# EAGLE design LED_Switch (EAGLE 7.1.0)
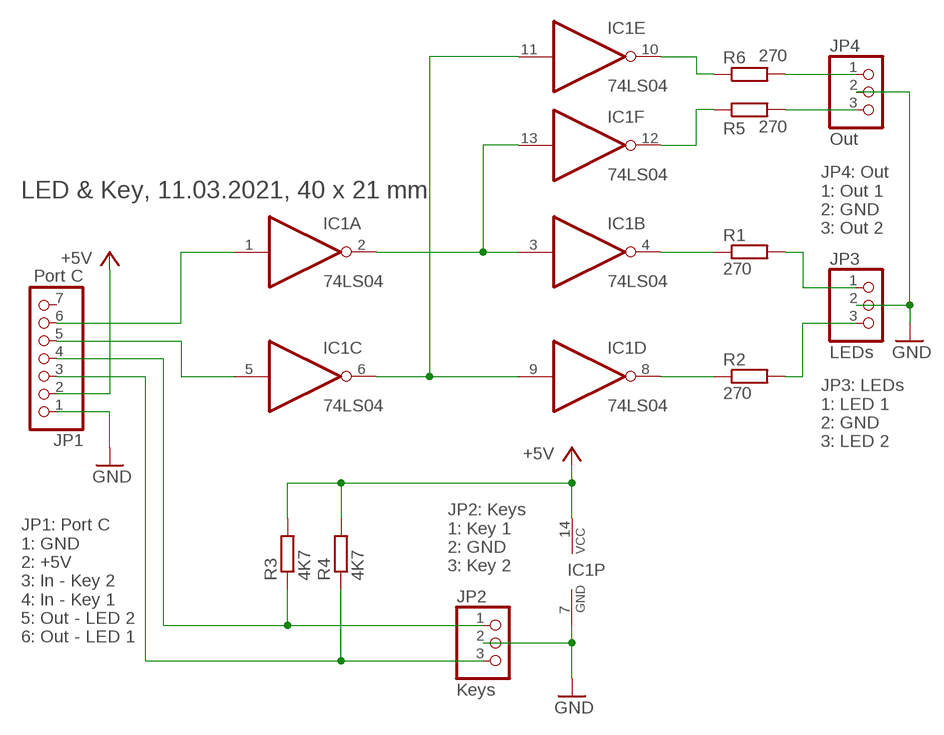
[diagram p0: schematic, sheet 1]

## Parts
IC1  74LS04  74ACT04D  [SO14]
JP1  Port C  PINHD-1X7  [1X07]
JP2  Keys  PINHD-1X3  [1X03]
JP3  LEDs  PINHD-1X3  [1X03]
JP4  Out  PINHD-1X3  [1X03]
R1  270  R-EU_R1206  [R1206]
R2  270  R-EU_R1206  [R1206]
R3  4K7  R-EU_R1206  [R1206]
R4  4K7  R-EU_R1206  [R1206]
R5  270  R-EU_R1206  [R1206]
R6  270  R-EU_R1206  [R1206]

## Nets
+5V: IC1.14(P:VCC) JP1.2 R3.2 R4.2
GND: IC1.7(P:GND) JP1.1 JP2.2 JP3.2 JP4.2
N$1: IC1.2(A:O) IC1.3(B:I) IC1.13(F:I)
N$2: IC1.6(C:O) IC1.9(D:I) IC1.11(E:I)
N$3: IC1.1(A:I) JP1.6
N$4: IC1.5(C:I) JP1.5
N$5: IC1.4(B:O) R1.1
N$6: IC1.8(D:O) R2.1
N$7: IC1.10(E:O) R6.1
N$8: JP3.1 R1.2
N$9: JP1.4 JP2.1 R3.1
N$10: JP1.3 JP2.3 R4.1
N$11: JP3.3 R2.2
N$12: IC1.12(F:O) R5.1
N$15: JP4.1 R6.2
N$16: JP4.3 R5.2
Unconnected: JP1.7

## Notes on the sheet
- LED & Key, 11.03.2021, 40 x 21 mm
- JP4: Out
  1: Out 1
  2: GND
  3: Out 2
- JP3: LEDs
  1: LED 1
  2: GND
  3: LED 2
- JP2: Keys
  1: Key 1
  2: GND
  3: Key 2
- JP1: Port C
  1: GND
  2: +5V
  3: In - Key 2
  4: In - Key 1
  5: Out - LED 2
  6: Out - LED 1

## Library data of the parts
IC1 = 74xx-eu:74*04: Hex INVERTER
JP1 = pinhead:PINHD-1X7: PIN HEADER
JP2-JP4 = pinhead:PINHD-1X3: PIN HEADER
R1-R6 = rcl:R-EU_: RESISTOR, European symbol

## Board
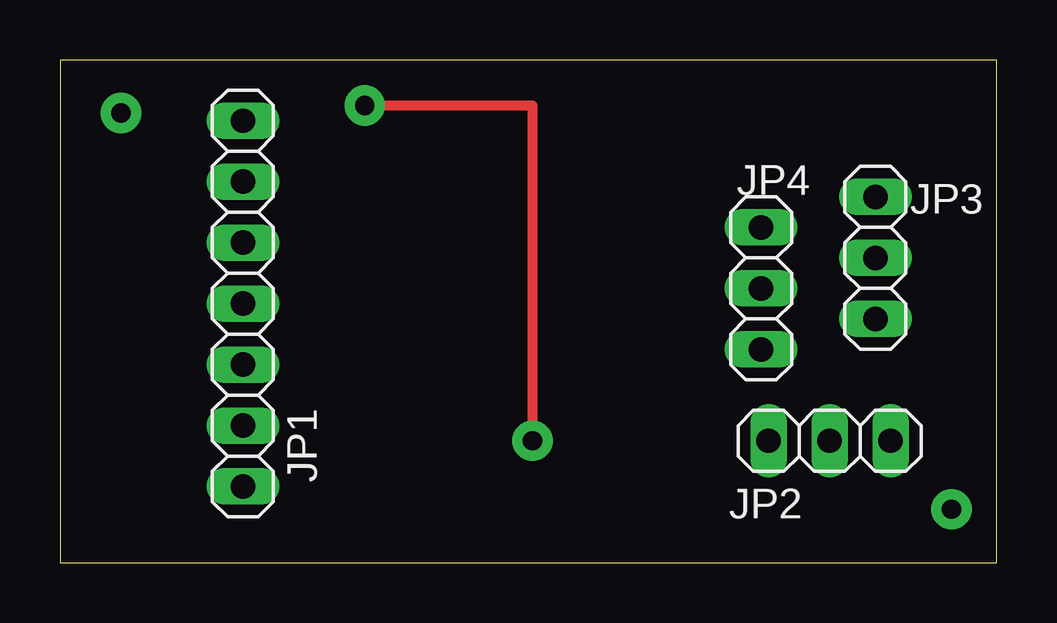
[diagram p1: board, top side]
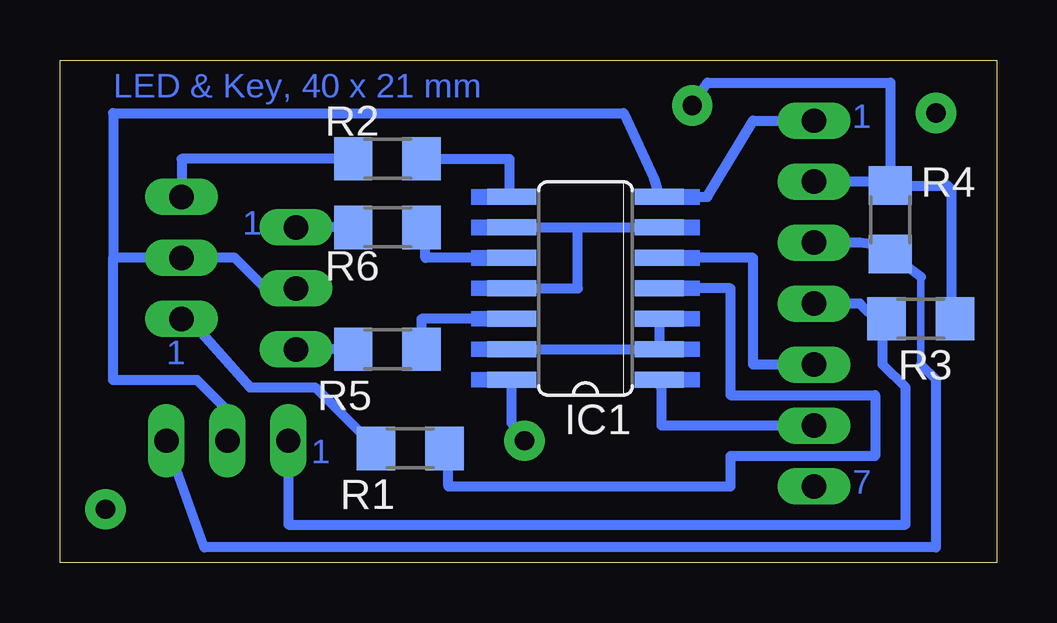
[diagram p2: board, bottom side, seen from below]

Size 39.04 x 20.95 mm. Coordinates in mm from the lower left corner, seen from the top.
Outline: 0,0 39.04,0 39.04,20.95 0,20.95 0,0
Copper layers (1*16): Top 0.035mm / dielectric 1.5mm / Bottom 0.035mm
Design rules "default": minimum track width 10mil, minimum drill 24mil, track to track 8mil, track to pad 8mil, pad to pad 8mil, via to via 8mil, smd to smd 8mil, copper to edge 40mil, drill to drill 8mil, minimum pad ring 10mil, minimum via ring 8mil, stop-mask expansion 4mil, vias tented up to drill 0mil, thermal gap 10mil

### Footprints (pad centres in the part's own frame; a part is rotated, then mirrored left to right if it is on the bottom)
SO14 = smd 0.66 x 2.032: 1 -3.81,-3.073; 2 -2.54,-3.073; 3 -1.27,-3.073; 4 0,-3.073; 5 1.27,-3.073; 6 2.54,-3.073; 7 3.81,-3.073; 8 3.81,3.073; 9 2.54,3.073; 10 1.27,3.073; 11 0,3.073; 12 -1.27,3.073; 13 -2.54,3.073; 14 -3.81,3.073
1X07 = drill 1.016 long: 1 -7.62,0; 2 -5.08,0; 3 -2.54,0; 4 0,0; 5 2.54,0; 6 5.08,0; 7 7.62,0
1X03 = drill 1.016 long: 1 -2.54,0; 2 0,0; 3 2.54,0
R1206 = smd 1.6 x 1.803: 1 -1.422,0; 2 1.422,0

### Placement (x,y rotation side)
IC1  17.14,11.43 90 bottom
JP1  7.62,10.79 270 top
JP2  32.07,5.08 0 top
JP3  33.97,12.7 90 top
JP4  29.21,11.43 270 top
R1  24.45,4.76 180 bottom
R2  25.4,16.83 180 bottom
R3  3.17,10.16 0 bottom
R4  4.45,14.29 90 bottom
R5  25.4,8.89 180 bottom
R6  25.4,13.97 180 bottom

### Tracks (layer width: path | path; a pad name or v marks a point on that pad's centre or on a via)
+5V  (via drill 0.8 pad 1.68)
  Top 0.406: v12.7,19.05 19.68,19.05 v19.68,5.08
  Bottom 0.406: R3.2 1.91,10.31 1.91,15.56 2.06,15.71 R4.2 4.45,15.88 | v19.68,5.08 20.22,5.82 IC1.14 | v12.7,19.05 12.06,20 4.45,20 4.45,15.88 | 4.45,15.88 JP1.2
GND
  Bottom 0.406: 36.83,12.7 JP3.2 31.75,12.7 30.48,11.43 JP4.2 | JP1.1 10.16,18.41 12.06,15.24 IC1.7 14.29,15.98 15.56,18.73 36.83,18.73 36.83,12.7 | 36.83,12.7 36.83,7.62 33.34,7.62 32.07,6.35 JP2.2
N$1
  Bottom 0.406: IC1.3 IC1.2 IC1.13
N$2
  Bottom 0.406: IC1.9 17.46,13.97 | 17.46,13.97 IC1.6 | IC1.11 17.46,11.43 17.46,13.97
N$3
  Bottom 0.406: 14.07,7.4 IC1.1 13.97,7.52 13.97,5.71 JP1.6
N$4
  Bottom 0.406: JP1.5 10.16,8.26 10.16,12.7 IC1.5
N$5
  Bottom 0.406: IC1.4 11.11,11.43 11.11,6.99 5.08,6.99 5.08,4.45 11.11,4.45 11.11,3.17 22.86,3.17 22.86,4.6 R1.1
N$6
  Bottom 0.406: IC1.8 20.32,15.24 20.32,16.83 R2.1
N$7
  Bottom 0.406: IC1.10 23.81,12.7 23.81,13.97 R6.1
N$8
  Bottom 0.406: JP3.1 33.66,10.16 31.11,7.3 28.41,7.3 R1.2
N$9
  Bottom 0.406: R3.1 4.45,10.16 | JP2.1 29.53,1.59 3.81,1.59 3.81,7.3 4.76,8.26 4.76,9.99 R3.1 | R3.1 4.92,9.99 5.71,10.79 JP1.4
N$10
  Bottom 0.305: 3.17,8.26 3.17,11.91
  Bottom 0.406: 3.17,8.26 2.54,7.62 2.54,0.64 33.02,0.64 JP2.3 | 3.17,11.91 R4.1 4.61,13.18 5.71,13.34 JP1.3
N$11
  Bottom 0.406: R2.2 33.97,16.83 JP3.3
N$12
  Bottom 0.406: IC1.12 23.98,10.16 R5.1
N$13  (via drill 0.8 pad 1.68)
  other vias: 2.54,18.73
N$14  (via drill 0.8 pad 1.68)
  other vias: 37.15,2.22
N$15
  Bottom 0.406: R6.2 JP4.1
N$16
  Bottom 0.406: R5.2 JP4.3
(copper drawn outside any net)
  shapes: Bottom area x14

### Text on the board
Bottom: LED & Key, 40 x 21 mm | 1 | 1 | 1 | 1 | 7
